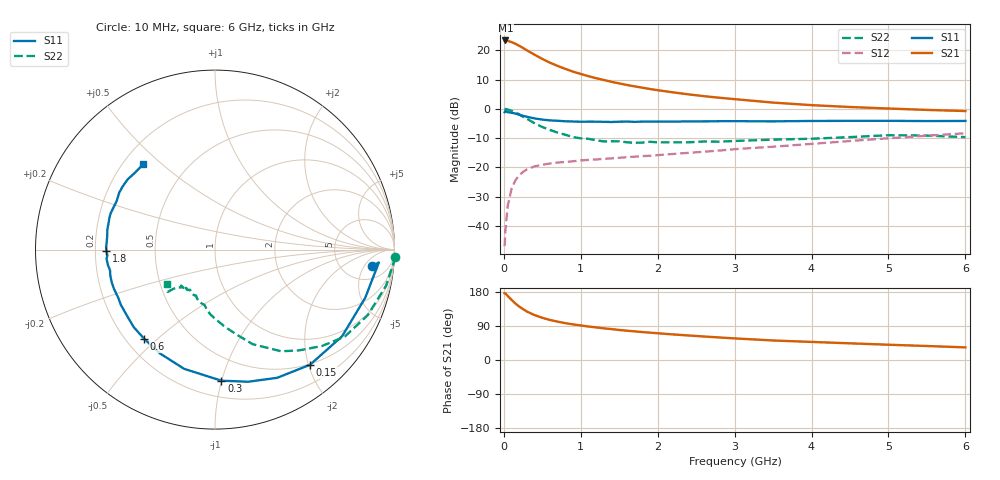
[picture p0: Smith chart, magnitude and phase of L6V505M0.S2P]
!  INFINEON TECHNOLOGIES Small Signal Semiconductors
! BFR380L3 , Si-NPN RF-Transistor in TSLP-3-1
!  Vce=0.5 V,  Ic=5 mA
! Common Emitter S-Parameters:  07. March 2005
#  GHz  S  MA  R  50
! f  S11  S21  S12  S22
! GHz  Mag  Ang  Mag  Ang  Mag  Ang  Mag  Ang
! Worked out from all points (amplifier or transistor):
!   36 points, 10 MHz to 6 GHz, reference 50 ohm
!   highest |S21| = 23.4 dB at 20 MHz (marker M1)
!   |S21| within 3 dB of that: start of sweep to 276.2 MHz
!   unconditionally stable (mu >= 1): 2.192 GHz to 5.543 GHz
!   at 250 MHz: K = 0.19, MSG = 21.2 dB, |S12| = -21.5 dB
!   at 1.4 GHz: K = 0.80, MSG = 13.1 dB, |S12| = -16.9 dB
!   at 6 GHz: K = 0.99, MSG = 3.8 dB, |S12| = -8.3 dB
!   S11 on the Smith chart (normalised r, x): 10 MHz: 9, -7; 150 MHz: 0.49, -2.03; 300 MHz: 0.32, -1.00; 600 MHz: 0.27, -0.45; 1.8 GHz: 0.25, -0.00; 6 GHz: 0.28, +0.43
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0.01  0.8771 -6.0  14.68 176.2  0.0045 84.5  1.006 -2.4
0.02  0.9158 -4.5  14.75 175.9  0.0084 86.0  0.9938 -5.1
0.05  0.879 -17.8  14.47 169.0  0.0218 80.1  0.9736 -12.0
0.1  0.8571 -34.3  13.82 158.8  0.0428 73.0  0.9264 -23.2
0.15  0.8318 -50.5  12.97 149.2  0.06 64.2  0.8702 -33.9
0.2  0.7939 -64.1  11.96 140.9  0.0733 58.5  0.8026 -42.0
0.25  0.7591 -75.9  10.97 134.2  0.0839 52.8  0.7302 -50.3
0.3  0.7312 -87.2  9.987 127.9  0.0924 49.0  0.6754 -57.0
0.4  0.6861 -104.5  8.403 118.4  0.1041 42.9  0.5672 -68.3
0.5  0.6551 -117.7  7.145 111.4  0.111 39.6  0.4892 -75.6
0.6  0.6348 -128.4  6.145 105.6  0.1163 37.4  0.4351 -82.5
0.8  0.6127 -143.6  4.818 97.2  0.1236 35.9  0.3606 -94.4
0.9  0.608 -149.9  4.322 94.0  0.1271 35.5  0.3294 -98.7
1.1  0.604 -158.5  3.614 88.3  0.1343 36.4  0.3072 -105.5
1.4  0.596 -168.7  2.896 81.6  0.1424 37.9  0.2796 -113.4
1.8  0.6056 -179.5  2.299 73.7  0.1556 41.3  0.2649 -122.2
2.2  0.6051 173.0  1.914 67.5  0.1694 44.3  0.268 -126.4
2.8  0.6146 163.1  1.549 59.5  0.1935 48.7  0.275 -133.3
3.5  0.6112 153.6  1.279 51.5  0.2255 51.3  0.2979 -135.0
4.5  0.6232 145.8  1.075 44.0  0.2819 54.5  0.3291 -137.2
5.5  0.6182 135.9  0.959 36.9  0.3475 53.9  0.3492 -140.5
6  0.6216 130.1  0.917 33.3  0.3829 52.6  0.3289 -144.6
